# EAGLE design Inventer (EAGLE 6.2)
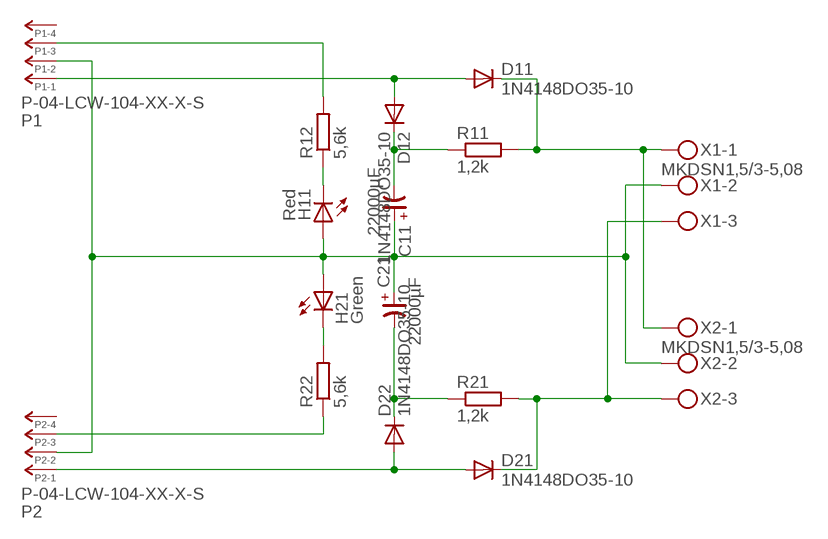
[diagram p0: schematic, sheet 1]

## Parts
C11  22000µF  CP-ETS-30  [ETS-30]
C21  22000µF  CP-ETS-30  [ETS-30]
D11  1N4148DO35-10  [DO35-10]
D12  1N4148DO35-10  [DO35-10]
D21  1N4148DO35-10  [DO35-10]
D22  1N4148DO35-10  [DO35-10]
H11  Red  LED5MM  [LED5MM]
H21  Green  LED5MM  [LED5MM]
P1  P-04-LCW-104-XX-X-S  [LCW-104-XX-X-S]
P2  P-04-LCW-104-XX-X-S  [LCW-104-XX-X-S]
R11  1,2k  R-EU_0207/12  [0207/12]
R12  5,6k  R-EU_0207/12  [0207/12]
R21  1,2k  R-EU_0207/12  [0207/12]
R22  5,6k  R-EU_0207/12  [0207/12]
X1  MKDSN1,5/3-5,08  [MKDSN1,5/3-5,08]
X2  MKDSN1,5/3-5,08  [MKDSN1,5/3-5,08]

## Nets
N$1: C11.+ C21.+ H11.A H21.A P1.2 P2.2 X1.2 X2.2
N$2: D11.C R11.2 X1.1 X2.1
N$3: D21.C R21.2 X1.3 X2.3
N$4: C11.- D12.C R11.1
N$5: D11.A D12.A P1.1
N$6: H11.K(C) R12.1
N$7: P1.3 R12.2
N$8: H21.K(C) R22.2
N$9: D21.A D22.A P2.1
N$10: P2.3 R22.1
N$11: C21.- D22.C R21.1
Unconnected: P1.4 P2.4

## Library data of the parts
C11 C21 = cap-master:CP-: POLARIZED CAP
D11 D12 D21 D22 = diode:1N4148: DIODE
H11 H21 = led:LED: LED
P1 P2 = con-headers-jp:P-04-: HEADER PLUG PINS
R11 R12 R21 R22 = resistor:R-EU_: RESISTOR, European symbol
X1 X2 = con-phoenix-508:MKDSN1,5/3-5,08: MKDSN 1,5/ 3-5,08 Printklemme Nennstrom: 13,5 A Nennspannung: 250 V Rastermaß: 5,08 mm Polzahl: 3 Anschlussart: Schraubanschluss Montage: Löten Anschlussrichtung Leiter/Platine: 0 ° Artikelnummer: 1729131 Source: http://eshop.phoenixcontact.com .. 1729131.pdf; MPN: SMKDSN1,5/3-5,08; OC_FARNELL: 1792904; OC_NEWARK: 70R0299

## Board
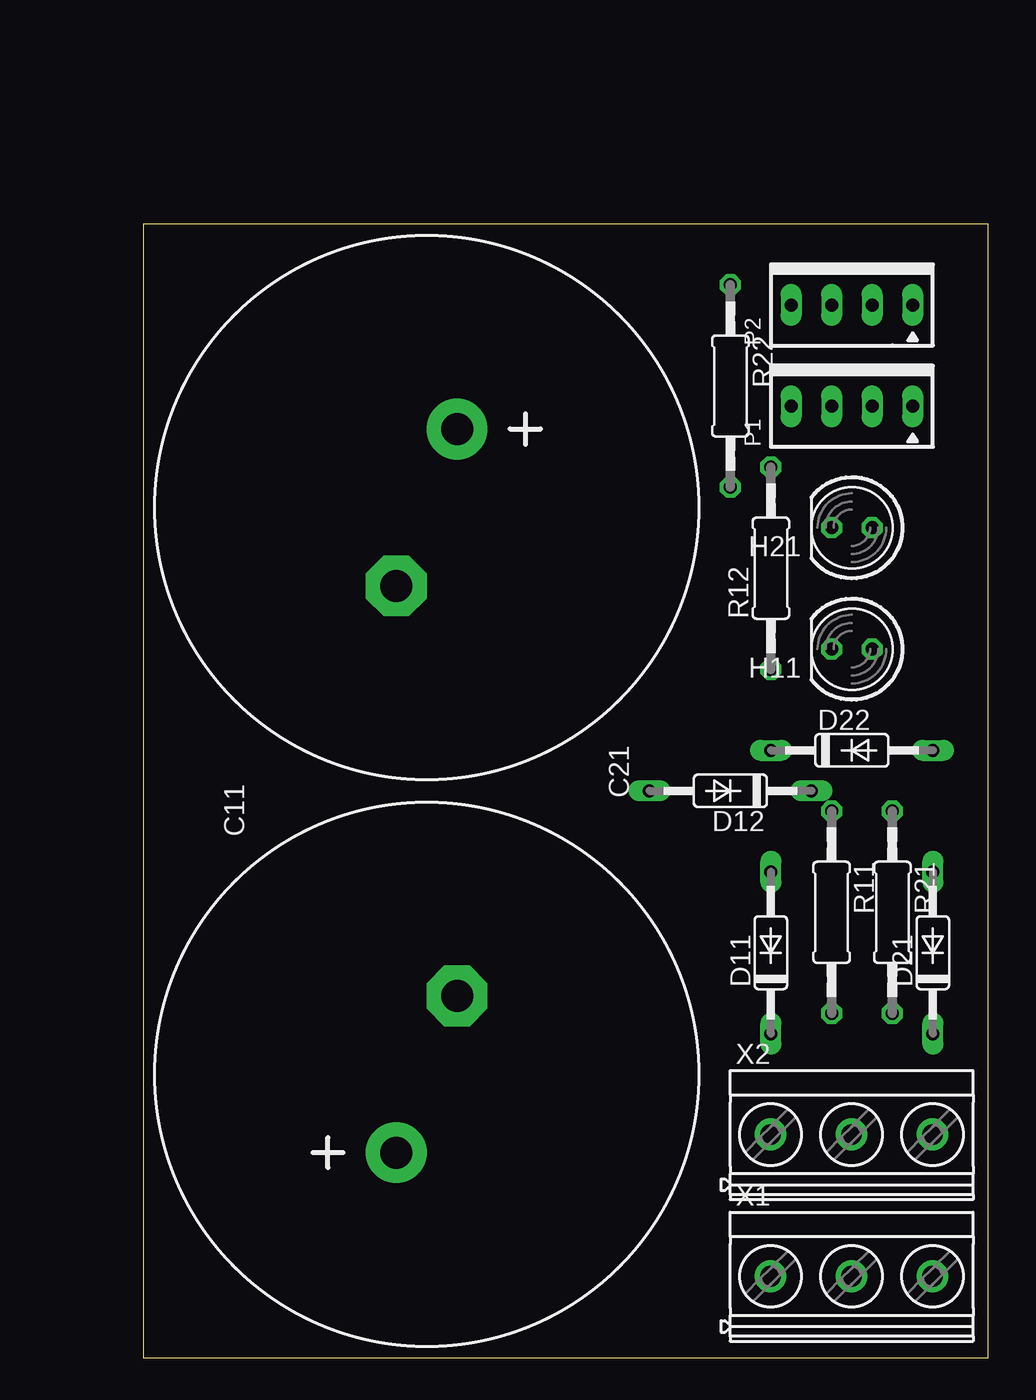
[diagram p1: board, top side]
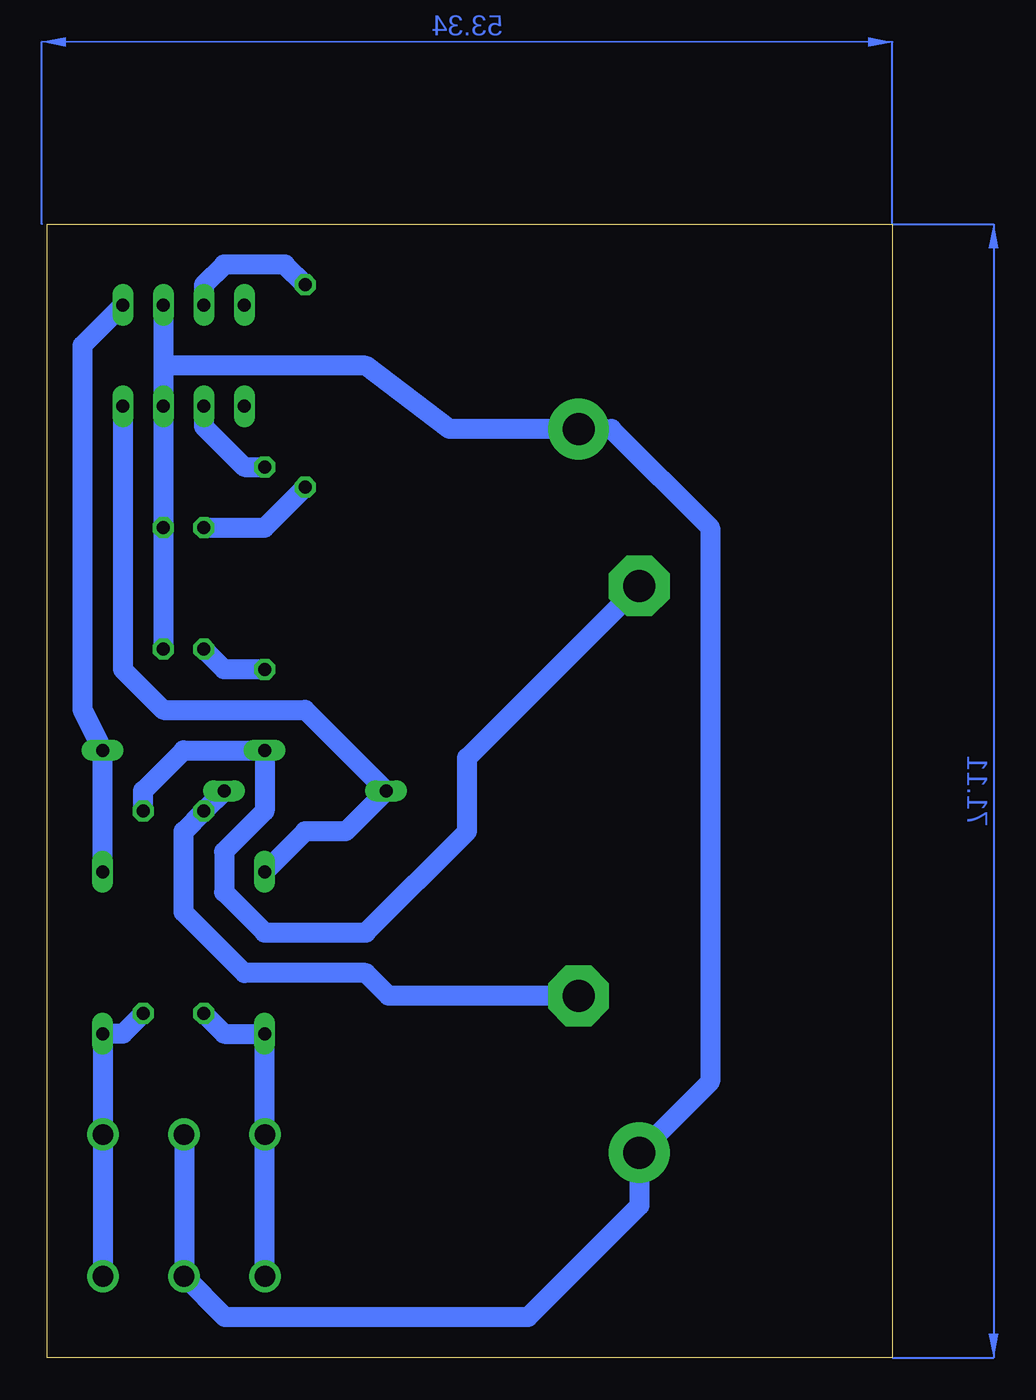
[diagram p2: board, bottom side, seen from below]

Size 53.01 x 71.11 mm. Coordinates in mm from the lower left corner, seen from the top.
Outline: 0,0 53.01,0 53.01,71.11 0,71.11 0,0
Copper layers (1*16): Top 0.035mm / dielectric 1.5mm / Bottom 0.035mm
Design rules: minimum track width 10mil, minimum drill 24mil, track to track 8mil, track to pad 8mil, pad to pad 8mil, via to via 8mil, smd to smd 8mil, copper to edge 40mil, drill to drill 8mil, minimum pad ring 10mil, minimum via ring 8mil, stop-mask expansion 4mil, vias tented up to drill 0mil, thermal gap 10mil

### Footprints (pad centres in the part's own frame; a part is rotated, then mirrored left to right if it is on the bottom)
ETS-30 = drill 2.007 pad 3.81: + -4.921,1.905 | drill 2.007 pad 3.81 octagon: - 4.921,-1.905
DO35-10 = drill 0.813 long: A 5.08,0; C -5.08,0
LED5MM = drill 0.813 octagon: A -1.27,0; K 1.27,0
LCW-104-XX-X-S = drill 0.813 long: 1 3.81,0; 2 1.27,0; 3 -1.27,0; 4 -3.81,0
0207/12 = drill 0.813 octagon: 1 -6.35,0; 2 6.35,0
MKDSN1,5/3-5,08 = drill 1.3 pad 2: 1 -7.641,0.025; 2 -2.561,0.025; 3 2.519,0.025

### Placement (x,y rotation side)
C11  17.78,17.78 90 top
C21  17.78,53.34 270 top
D11  39.37,25.4 90 top
D12  36.83,35.56 180 top
D21  49.53,25.4 90 top
D22  44.45,38.1 0 top
H11  44.45,44.45 180 top
H21  44.45,52.07 180 top
P1  44.45,59.69 0 top
P2  44.45,66.04 0 top
R11  43.18,27.94 270 top
R12  39.37,49.53 90 top
R21  46.99,27.94 270 top
R22  36.83,60.96 270 top
X1  46.99,5.08 0 top
X2  46.99,13.97 0 top

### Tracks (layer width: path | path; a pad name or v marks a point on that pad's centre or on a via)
N$1
  Bottom 1.27: X2.2 X1.2 41.86,2.54 22.86,2.54 15.88,9.53 C11.+ 11.43,17.3 11.43,52.07 17.62,58.26 C21.+ 27.78,58.26 33.02,62.23 45.72,62.23 | P2.2 45.72,62.23 | 45.72,62.23 P1.2 H21.A H11.A
N$2
  Bottom 0.406: 39.35,20.3 D11.C
  Bottom 1.27: X1.1 X2.1 39.35,20.3 | R11.2 41.91,20.32 D11.C
N$3
  Bottom 0.406: 49.53,14.02 X2.3
  Bottom 1.27: X1.3 X2.3 | 49.53,14.02 D21.C 48.26,20.32 R21.2
N$4
  Bottom 1.27: D12.C R11.1 44.45,33.02 44.45,27.94 40.64,24.13 33.02,24.13 31.59,22.7 C11.-
N$5
  Bottom 1.27: D11.A 36.83,33.02 34.29,33.02 D12.A 36.83,40.64 45.72,40.64 48.26,43.18 P1.1
N$6
  Bottom 1.27: R12.1 41.91,43.18 H11.K
N$7
  Bottom 1.27: P1.3 43.18,58.42 40.64,55.88 R12.2
N$8
  Bottom 1.27: H21.K 39.37,52.07 R22.2
N$9
  Bottom 1.27: P2.1 50.8,63.5 50.8,40.64 D22.A D21.A
N$10
  Bottom 1.27: R22.1 38.1,68.58 41.91,68.58 43.18,67.31 P2.3
N$11
  Bottom 1.27: C21.- 26.67,37.62 26.67,33.02 33.02,26.67 39.37,26.67 41.91,29.21 41.91,31.75 39.37,34.29 D22.C 44.45,38.1 46.99,35.56 R21.1
(copper drawn outside any net)
  shapes: Bottom area x2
